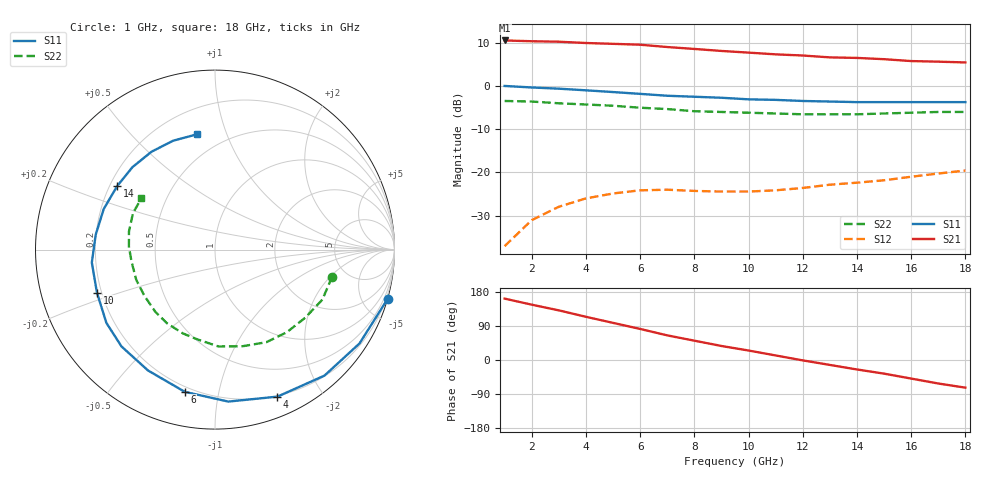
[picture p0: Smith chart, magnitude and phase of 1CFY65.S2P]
!CFY65, AlGaAs/GaAs HEMT in CEREC-XF package
!V ds = 2V, I d = 10mA
# GHZ S MA R 50
!f GHz  S11  S21  S12  S22
!  MAG  ANG  MAG  ANG  MAG  ANG  MAG  ANG
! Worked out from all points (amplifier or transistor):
!   18 points, 1 GHz to 18 GHz, reference 50 ohm
!   highest |S21| = 10.5 dB at 1 GHz (marker M1)
!   |S21| within 3 dB of that: start of sweep to 10.46 GHz
!   unconditionally stable (mu >= 1): 8.68 GHz to 16.41 GHz
!   at 4 GHz: K = 0.47, MSG = 18.0 dB, |S12| = -26.0 dB
!   at 10 GHz: K = 1.17, MAG = 13.6 dB, |S12| = -24.4 dB
!   at 18 GHz: K = 0.89, MSG = 12.5 dB, |S12| = -19.6 dB
!   lowest NFmin = 0.40 dB at 4 GHz
!   S11 on the Smith chart (normalised r, x): 1 GHz: -0.00, -7.12; 4 GHz: 0.19, -1.49; 6 GHz: 0.17, -0.80; 10 GHz: 0.18, -0.17; 14 GHz: 0.23, +0.28; 18 GHz: 0.36, +0.79
1  1 -16.0  3.36 162.0  0.014 77.0  0.67 -13.0
2  0.96 -33.0  3.29 146.0  0.028 65.0  0.66 -25.0
3  0.93 -49.0  3.25 131.0  0.04 55.0  0.63 -37.0
4  0.89 -67.0  3.14 114.0  0.05 43.0  0.61 -49.0
5  0.85 -85.0  3.07 98.0  0.057 35.0  0.59 -61.0
6  0.81 -102.0  3 82.0  0.062 25.0  0.56 -74.0
7  0.77 -119.0  2.82 65.0  0.063 16.0  0.54 -88.0
8  0.75 -134.0  2.68 51.0  0.061 8.0  0.51 -101.0
9  0.73 -146.0  2.54 37.0  0.06 6.0  0.5 -111.0
10  0.7 -160.0  2.43 25.0  0.06 5.0  0.49 -123.0
11  0.69 -174.0  2.32 12.0  0.062 4.0  0.48 -134.0
12  0.67 173.0  2.25 -1.0  0.066 3.0  0.47 -147.0
13  0.66 160.0  2.14 -13.0  0.072 0.0  0.47 -159.0
14  0.65 147.0  2.11 -25.0  0.076 -5.0  0.47 -172.0
15  0.65 135.0  2.04 -36.0  0.081 -8.0  0.48 178.0
16  0.65 123.0  1.94 -49.0  0.089 -13.0  0.49 168.0
17  0.65 111.0  1.91 -62.0  0.097 -19.0  0.5 156.0
18  0.65 99.0  1.87 -73.0  0.105 -26.0  0.5 145.0
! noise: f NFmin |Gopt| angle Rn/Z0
4  0.4  0.66  69  0.27
6  0.51  0.6  106  0.18
8  0.66  0.56  138  0.102
10  0.86  0.53  170  0.066
12  1.07  0.46  -163  0.058
14  1.25  0.44  -136  0.054
